(* Logix 5000 AddOnInstructionDefinition export AMCI_MA_Registration_Move; software revision 20.05 *)

TYPE AMCI_Motion_Axis_Output_Data :
STRUCT
   Control_Word_0 : INT;
   Control_Word_1 : INT;
   Position_or_Distance : DINT;
   Programmed_Speed : DINT;
   Acceleration : INT;
   Deceleration : INT;
   Output_Word_8 : INT;
   Output_Word_9 : INT;
END_STRUCT
END_TYPE

TYPE AMCI_Motion_Axis_Input_Data :
STRUCT
   Moving_CW : BOOL;
   Moving_CCW : BOOL;
   In_Hold_State : BOOL;
   Stopped : BOOL;
   At_Home : BOOL;
   Accelerating : BOOL;
   Decelerating : BOOL;
   Move_Complete : BOOL;
   Status_Word_0_Bit_8 : BOOL;
   Status_Word_0_Bit_9 : BOOL;
   Position_Invalid : BOOL;
   Input_Error : BOOL;
   Command_Error : BOOL;
   Configuration_Error : BOOL;
   Module_OK : BOOL;
   Mode_Flag : BOOL;
   IN1_Active : BOOL;
   IN2_Active : BOOL;
   IN3_Active : BOOL;
   IN4_Active : BOOL;
   Status_Word_1_Bit_4 : BOOL;
   Status_Word_1_Bit_5 : BOOL;
   Connection_Was_Lost : BOOL;
   Driver_Fault : BOOL;
   Status_Word_1_Bit_8 : BOOL;
   Invalid_Jog_Change : BOOL;
   Status_Word_1_Bit_10 : BOOL;
   Heartbeat_Bit : BOOL;
   Status_Word_1_Bit_12 : BOOL;
   Status_Word_1_Bit_13 : BOOL;
   Stall_Detected : BOOL;
   Drive_Is_Enabled : BOOL;
   Motor_Position : DINT;
   Encoder_Position : DINT;
   Trapped_Encoder_Position : DINT;
   Input_Word_8 : INT;
   Input_Word_9 : INT;
END_STRUCT
END_TYPE

ADD_ON_INSTRUCTION AMCI_MA_Registration_Move   (* revision 1.0, vendor AMCI, ExecuteEnableInFalse *)
// AMCI Motion Axis Registration Move
// Revision note:
// 12/01/2022 Initial release of AOI.
// Help:
// MOTION AXIS REGISTRATION MOVE
// AXIS INPUT DATA:  Input data from AMCI motion device.   Uses the AMCI_Motion_Axis_Input_Data User Defined Data Type.
// AXIS OUTPUT DATA; Output data from the AOI to the AMCI motion device.   Uses the AMCI_Motion_Axis_Output_Data User Defined Data Type.
// DIRECTION: 0 = CW motion 1 = CCW motion
// STOPPING_DISTANCE: The number of steps to move after the registration input has become active.
// PROGRAMMED SPEED: Speed of move in units of steps / sec
// ACCELERATION: Acceleration Rate in units of steps / sec / ms
// DECELERATION:  Deceleration Rate in units of steps / sec / ms
// MINIMUM REGISTRATION DISTANCE: The number of steps to move during which the registration input is                                                                   ignored.
// EN (Enable) Set when rung is true, Reset when rung is false
// DN (Done) Set when command is sent to the motion device.  Reset when the rung is false.
// ER (Error) Set when a command or input error failed to clear.  Reset when the rung is false.
// IP (In Process) Set when motion is occurring.   Reset when motion stops or the rung goes false.
VAR_IN_OUT
   Axis_Input_Data : AMCI_Motion_Axis_Input_Data; {required}
        [0].6   // set when decelerating
   Axis_Output_Data : AMCI_Motion_Axis_Output_Data; {required}
END_VAR
VAR_INPUT
   Direction_0_CW_1_CCW : BOOL; {required}   // 0=jog CW 1=jog CCW
   Stopping_Distance : DINT; {required}
   Programmed_Speed : DINT; {required}
   Acceleration : INT; {required}
   Deceleration : INT; {required}
   Minimum_Registration_Distance : DINT; {required}
END_VAR
VAR_OUTPUT
   EN : BOOL; {visible}   // set when rung with AOI is true
   DN : BOOL; {access Read Only, visible}   // set when move was succesfully initiated
   ER : BOOL; {visible}
   IP : BOOL; {visible}   // set when motion occurring
END_VAR
VAR
   command_data_block : INT[10];
        [0]   // Command Bits MSW
        [1]   // Command Bits LSW
        [2]   // Upper Target Position
        [3]   // Lower Target Position
        [4]   // Upper Programmed Speed
        [5]   // Lower Programmed Speed
   motion_occurring : BOOL; {access None}
   Internal_Enable : BOOL; {access None}   // set when driver ready to receive motion command
END_VAR

ROUTINE EnableInFalse   (* ladder *)
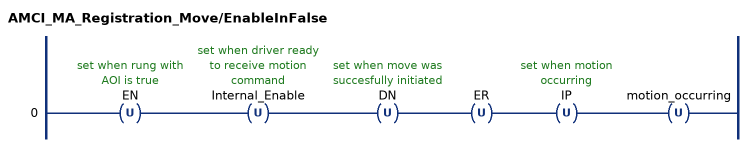
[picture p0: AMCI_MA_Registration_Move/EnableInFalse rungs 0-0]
   0: OTU(EN)OTU(Internal_Enable)OTU(DN)OTU(ER)OTU(IP)OTU(motion_occurring);
END_ROUTINE

ROUTINE Logic   (* ladder *)
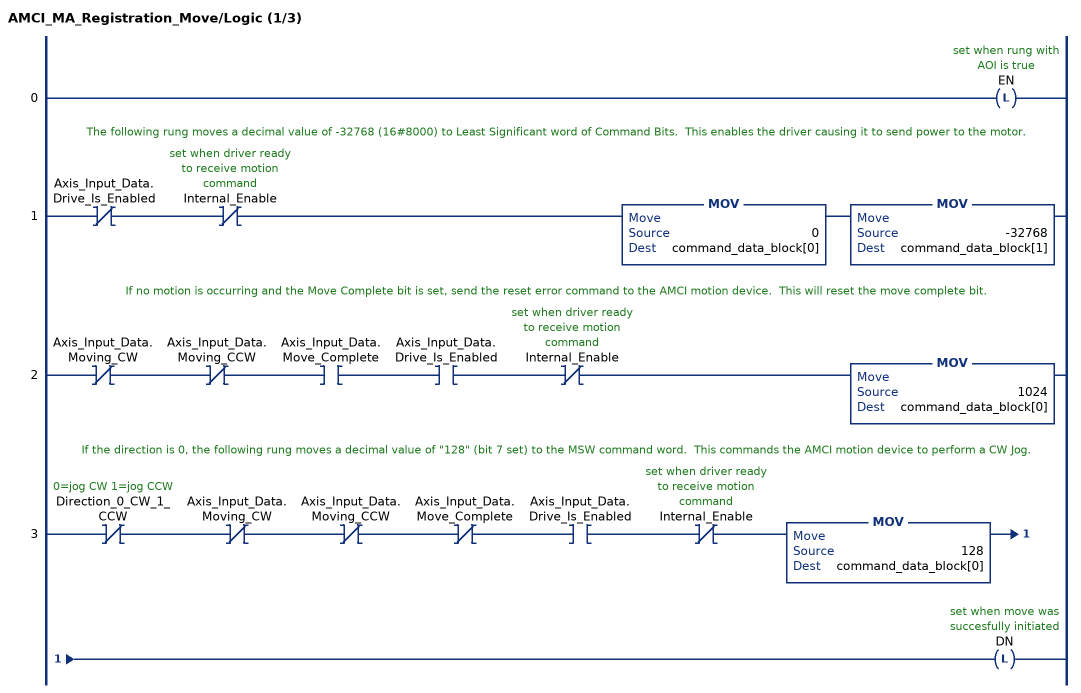
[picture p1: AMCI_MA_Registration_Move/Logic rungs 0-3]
   0: OTL(EN);
   // The following rung moves a decimal value of -32768 (16#8000) to Least Significant word of Command Bits.  This enables the driver causing it to send power to the motor.
   1: XIO(Axis_Input_Data.Drive_Is_Enabled)XIO(Internal_Enable)MOV(0,command_data_block[0])MOV(-32768,command_data_block[1]);
   // If no motion is occurring and the Move Complete bit is set, send the reset error command to the AMCI motion device.  This will reset the move complete bit.
   2: XIO(Axis_Input_Data.Moving_CW)XIO(Axis_Input_Data.Moving_CCW)XIC(Axis_Input_Data.Move_Complete)XIC(Axis_Input_Data.Drive_Is_Enabled)XIO(Internal_Enable)MOV(1024,command_data_block[0]);
   // If the direction is 0, the following rung moves a decimal value of "128" (bit 7 set) to the MSW command word.  This commands the AMCI motion device to perform a CW Jog.
   3: XIO(Direction_0_CW_1_CCW)XIO(Axis_Input_Data.Moving_CW)XIO(Axis_Input_Data.Moving_CCW)XIO(Axis_Input_Data.Move_Complete)XIC(Axis_Input_Data.Drive_Is_Enabled)XIO(Internal_Enable)MOV(128,command_data_block[0])OTL(DN);
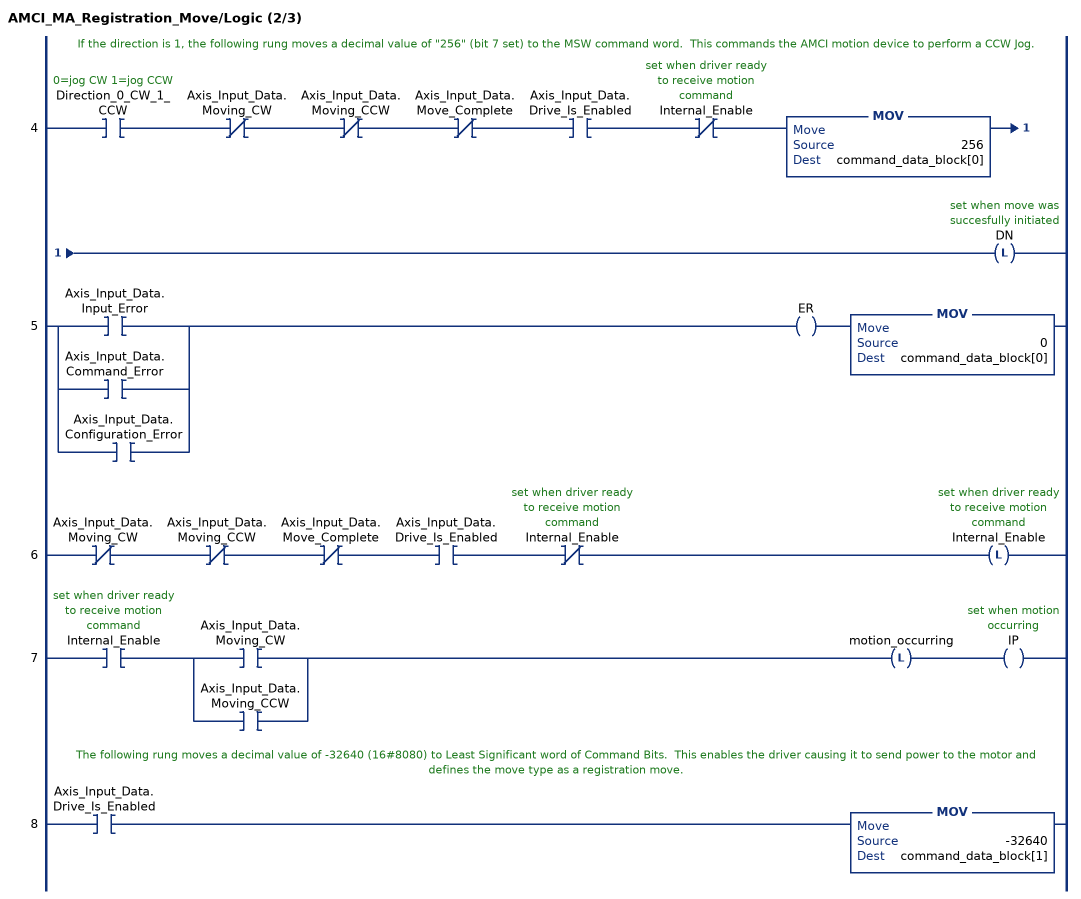
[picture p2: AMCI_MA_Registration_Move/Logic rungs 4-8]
   // If the direction is 1, the following rung moves a decimal value of "256" (bit 7 set) to the MSW command word.  This commands the AMCI motion device to perform a CCW Jog.
   4: XIC(Direction_0_CW_1_CCW)XIO(Axis_Input_Data.Moving_CW)XIO(Axis_Input_Data.Moving_CCW)XIO(Axis_Input_Data.Move_Complete)XIC(Axis_Input_Data.Drive_Is_Enabled)XIO(Internal_Enable)MOV(256,command_data_block[0])OTL(DN);
   5: [XIC(Axis_Input_Data.Input_Error) ,XIC(Axis_Input_Data.Command_Error) ,XIC(Axis_Input_Data.Configuration_Error) ]OTE(ER)MOV(0,command_data_block[0]);
   6: XIO(Axis_Input_Data.Moving_CW)XIO(Axis_Input_Data.Moving_CCW)XIO(Axis_Input_Data.Move_Complete)XIC(Axis_Input_Data.Drive_Is_Enabled)XIO(Internal_Enable)OTL(Internal_Enable);
   7: XIC(Internal_Enable)[XIC(Axis_Input_Data.Moving_CW) ,XIC(Axis_Input_Data.Moving_CCW) ]OTL(motion_occurring)OTE(IP);
   // The following rung moves a decimal value of -32640 (16#8080) to Least Significant word of Command Bits.  This enables the driver causing it to send power to the motor and defines the move type as a registration move.
   8: XIC(Axis_Input_Data.Drive_Is_Enabled)MOV(-32640,command_data_block[1]);
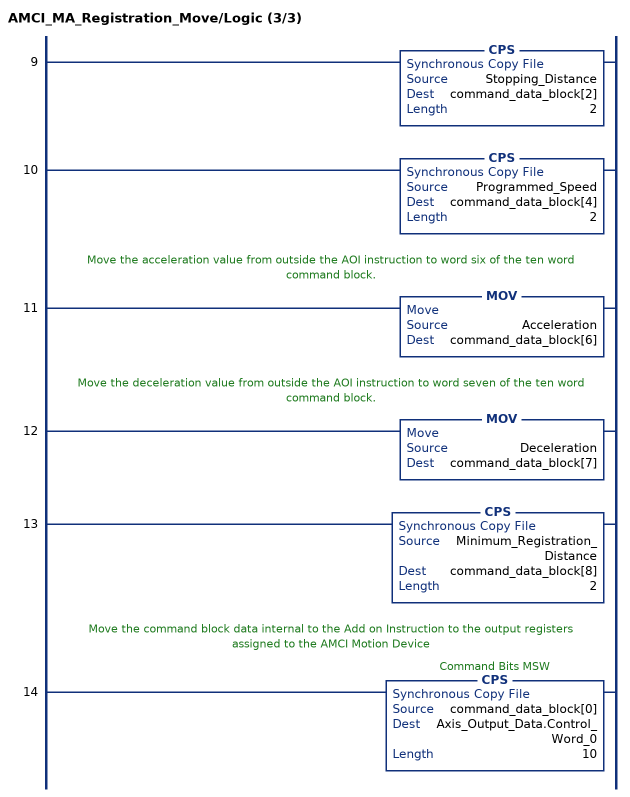
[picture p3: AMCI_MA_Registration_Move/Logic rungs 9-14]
   9: CPS(Stopping_Distance,command_data_block[2],2);
   10: CPS(Programmed_Speed,command_data_block[4],2);
   // Move the acceleration value from outside the AOI instruction to word six of the ten word command block.
   11: MOV(Acceleration,command_data_block[6]);
   // Move the deceleration value from outside the AOI instruction to word seven of the ten word command block.
   12: MOV(Deceleration,command_data_block[7]);
   13: CPS(Minimum_Registration_Distance,command_data_block[8],2);
   // Move the command block data internal to the Add on Instruction to the output registers assigned to the AMCI Motion Device
   14: CPS(command_data_block[0],Axis_Output_Data.Control_Word_0,10);
END_ROUTINE
END_ADD_ON_INSTRUCTION
